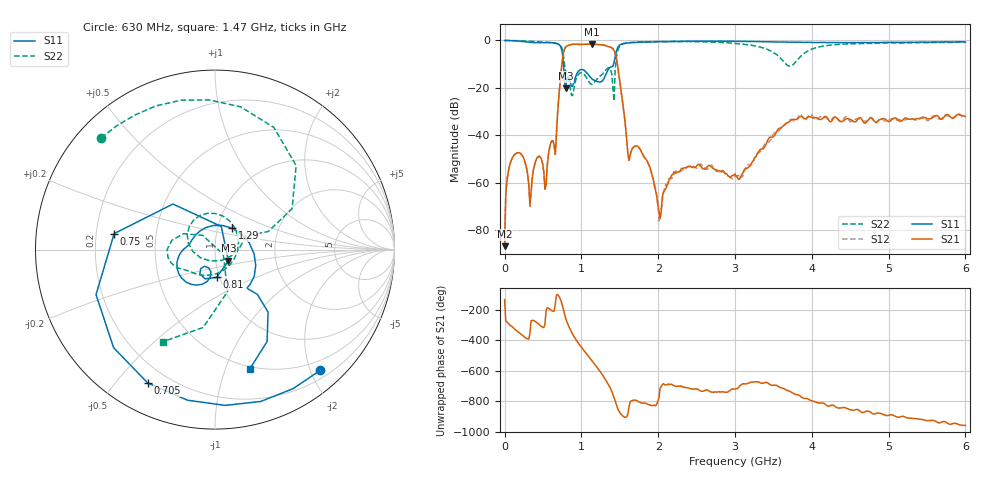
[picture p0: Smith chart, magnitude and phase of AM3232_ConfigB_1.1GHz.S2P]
! Network Analyzer HP8753E.07.74: Oct 30, 2002 Serial No. US37390186
! 24 Jul 2023  07:16:30
! Frequency  S11  S21  S12  S22
# HZ  S  DB R  50
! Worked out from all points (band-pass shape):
!   401 points, 30 kHz to 6 GHz, reference 50 ohm
!   highest |S21| = -1.53 dB at 1.14 GHz (marker M1); lowest = -86.8 dB at 30 kHz (marker M2)
!   |S21| within 3 dB of the highest: 772.9 MHz to 1.429 GHz (656.3 MHz wide, 59.6 % of centre)
!   lowest |S11| = -20.3 dB at 795 MHz (marker M3), VSWR 1.21, Z = 57.6 - j7.18 ohm
!   |S11| at or under -10 dB: 766.4 MHz to 1.418 GHz (651.5 MHz wide, 59.7 % of centre)
!   |S22| runs from -25.5 to 0.0 dB; largest |S21 - S12| = 0.032
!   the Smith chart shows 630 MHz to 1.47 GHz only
!   S11 on the Smith chart (normalised r, x): 630 MHz: 0.33, -2.15; 705 MHz: 0.13, -0.61; 750 MHz: 0.28, +0.07; 810 MHz: 0.97, -0.31; 1.29 GHz: 1.17, +0.29; 1.47 GHz: 0.48, -1.22
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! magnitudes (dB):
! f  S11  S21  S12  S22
! 30 kHz  0.0  -86.8  -82.5  0.0
! 120 MHz  -0.1  -48.5  -48.5  0.0
! 330 MHz  -0.8  -70.1  -68.7  -0.3
! 630 MHz  -1.0  -42.3  -42.3  -1.0
! 705 MHz  -1.6  -24.2  -24.0  -1.6
! 750 MHz  -4.9  -8.8  -8.7  -3.7
! 795 MHz  -20.3  -2.8  -2.7  -13.2
! 810 MHz  -16.2  -2.4  -2.3  -14.5
! 1.005 GHz  -12.2  -1.7  -1.7  -13.7
! 1.14 GHz  -16.3  -1.5  -1.6  -18.5
! 1.29 GHz  -16.3  -1.9  -2.0  -13.7
! 1.41 GHz  -10.8  -3.4  -3.6  -19.6
! 1.47 GHz  -3.2  -10.3  -10.2  -4.6
! 1.62 GHz  -1.0  -50.7  -50.6  -0.9
! 1.86 GHz  -0.6  -51.1  -51.2  -0.6
! 2.01 GHz  -0.5  -71.9  -76.2  -0.4
! 2.25 GHz  -0.4  -55.5  -54.7  -0.4
! 3 GHz  -0.3  -56.3  -57.2  -1.2
! 3.705 GHz  -0.7  -34.3  -33.8  -10.8
! 4.005 GHz  -0.8  -32.5  -31.7  -3.6
! 5.01 GHz  -0.8  -34.3  -33.5  -1.0
! 6 GHz  -0.7  -32.0  -32.2  -0.7
